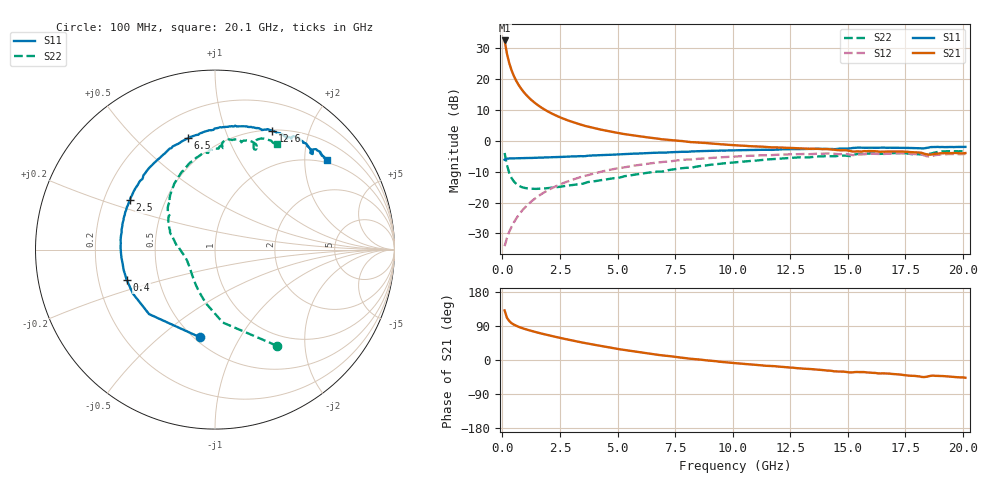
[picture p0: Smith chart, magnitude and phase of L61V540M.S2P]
!  Infineon Technologies AG
! BFR380L3 , PF131585-7, No.6, Th 09.10.01, soldered on pcb-board, measured with PP GSG850
!  Vce=1.5 V,  Ic=40.0 mA
! Common Emitter S-Parameters:  15. November 2001
#  GHz  S  MA  R  50
! f  S11  S21  S12  S22
! GHz  Mag  Ang  Mag  Ang  Mag  Ang  Mag  Ang
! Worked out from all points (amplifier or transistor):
!   201 points, 100 MHz to 20.1 GHz, reference 50 ohm
!   highest |S21| = 32.6 dB at 100 MHz (marker M1)
!   |S21| within 3 dB of that: start of sweep to 170.4 MHz
!   unconditionally stable (mu >= 1): 943.5 MHz to 4.52 GHz
!   at 3.4 GHz: K = 1.02, MAG = 7.7 dB, |S12| = -11.7 dB
!   at 10.1 GHz: K = 0.97, MSG = 1.8 dB, |S12| = -5.1 dB
!   at 20.1 GHz: K = 0.99, MSG = 0.1 dB, |S12| = -4.2 dB
!   S11 on the Smith chart (normalised r, x): 100 MHz: 0.53, -0.69; 400 MHz: 0.32, -0.15; 2.5 GHz: 0.31, +0.25; 6.5 GHz: 0.35, +0.73; 12.6 GHz: 0.51, +1.47; 20.1 GHz: 0.93, +2.57
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0.1  0.4953 -99.9  42.7 130.8  0.01957 59.5  0.6372 -57.2
0.2  0.514 -135.6  26.15 111.6  0.02645 56.5  0.4085 -83.9
0.3  0.5188 -151.7  18.36 102.8  0.03369 59.1  0.304 -99.5
0.4  0.5202 -160.9  14.06 97.3  0.0402 61.9  0.2507 -110.8
0.5  0.5212 -167.2  11.35 93.4  0.04737 64.3  0.2204 -119.7
0.6  0.5207 -171.7  9.511 90.4  0.05469 66.0  0.2014 -126.6
0.7  0.5232 -175.4  8.19 87.7  0.06192 66.8  0.1893 -132.6
0.8  0.5245 -178.6  7.189 85.4  0.06942 67.9  0.181 -137.5
1  0.5262 176.1  5.787 81.4  0.08447 68.5  0.1718 -145.3
1.3  0.5293 169.7  4.483 76.1  0.1073 68.3  0.1671 -153.8
1.6  0.5353 164.1  3.671 71.3  0.13 67.3  0.1674 -159.9
2  0.5416 157.4  2.972 65.4  0.1598 65.2  0.1716 -166.3
2.5  0.5486 149.8  2.42 58.4  0.1962 62.1  0.1801 -172.8
3.5  0.5642 135.9  1.793 45.7  0.2663 55.0  0.2018 176.8
4.9  0.6005 119.5  1.374 30.4  0.3532 44.8  0.2494 162.2
6.5  0.6392 103.5  1.12 15.7  0.4365 33.1  0.3106 146.8
6.8  0.6442 100.8  1.083 13.2  0.4498 30.8  0.3183 143.8
10.1  0.7055 76.9  0.8502 -8.1  0.5584 9.2  0.4501 117.5
12.6  0.735 64.2  0.7673 -20.2  0.6079 -5.7  0.5315 99.0
13.5  0.7403 60.0  0.7471 -24.5  0.6159 -10.7  0.5502 93.5
16.8  0.775 47.7  0.6738 -35.8  0.6197 -26.0  0.6307 74.5
20.1  0.7996 38.5  0.6354 -46.8  0.6142 -39.3  0.6834 59.4
